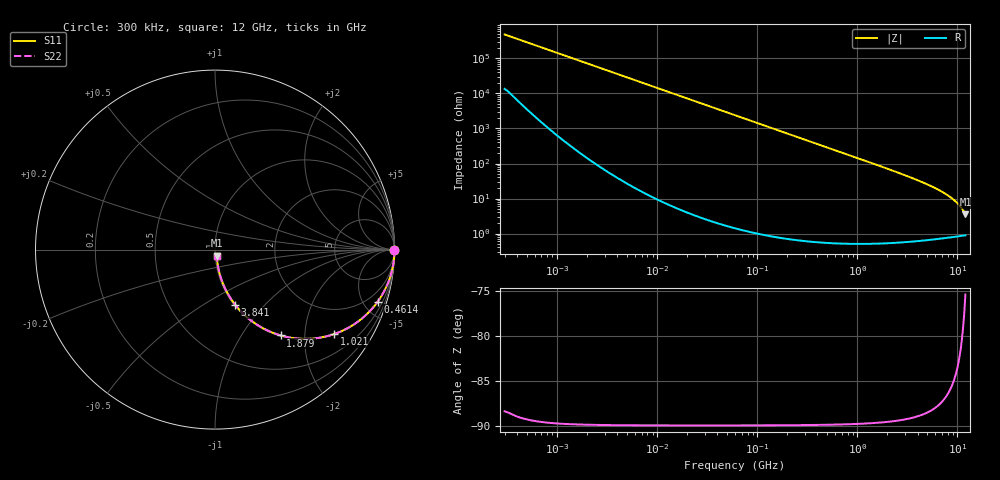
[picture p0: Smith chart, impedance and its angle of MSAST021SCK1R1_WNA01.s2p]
! MSAST021SCK1R1_WNA01  S-PARAMETER MODEL  ( General Type )
! Model Generated by TAIYO YUDEN Corporation (http://www.ty-top.com)
! Version 2.0
! TAIYO YUDEN Control No. 181101
! Copyright(c) 2015 TAIYO YUDEN CO.,LTD. All Rights Reserved.
! Product Description (link to TY-COMPAS)
! https://ds.yuden.co.jp/TYCOMPAS/or/detail?pn=MSAST021SCK1R1BWNA01&u=M
! Products Name : Multilayer Ceramic Capacitors
! Characteristics :
!  Capacitance : 1.1 pF , Rated Voltage : 25V , TCC : CK / C0K
!  Case Size : 0.25 x 0.125 / 0.0098 x 0.0049 [mm/inch] , Thickness : 0.125 / 0.0049 [mm/inch]
!  (Conditions: Temperature = 25 degC , DC Bias Current/Voltage = 0A / 0V)
! External Node Assignments :
!  1  o---| |---o  2
! GND o---------o GND
! Frequency Range : 0.3MHz  -  12000MHz  [ 401 STEP ]
# MHz S RI R 50
! Freq[MHz].  S11 Real  S11 Imag  S21 Real  S21 Imag  S12 Real  S12 Imag  S22 Real  S22 Imag
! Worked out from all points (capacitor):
!   401 points, 300 kHz to 12 GHz, reference 50 ohm
!   read as one part in series: C = 1.1 pF near 316.3 kHz
!   lowest |Z| = 3.54 ohm at 12 GHz (marker M1)
!   S11 on the Smith chart (normalised r, x): 300 kHz: open; 461.4 MHz: 1.01, -6.27; 1.021 GHz: 1.01, -2.82; 1.879 GHz: 1.01, -1.51; 3.841 GHz: 1.01, -0.70; 12 GHz: 1.02, -0.07
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0.3  1 -0.000207  5.83e-06 0.000207  5.83e-06 0.000207  1 -0.000207
1.769972  1 -0.00122  4.23e-06 0.00122  4.23e-06 0.00122  1 -0.00122
10.44266  0.9999 -0.00722  5.67e-05 0.00722  5.67e-05 0.00722  0.9999 -0.00722
60  0.9983 -0.0414  0.00174 0.0414  0.00174 0.0414  0.9983 -0.0414
159.8975  0.9878 -0.1092  0.0122 0.1092  0.0122 0.1092  0.9878 -0.1092
237.9135  0.9735 -0.1601  0.0265 0.1601  0.0265 0.1601  0.9735 -0.1601
353.9943  0.9432 -0.2308  0.0568 0.2308  0.0568 0.2308  0.9432 -0.2308
461.3684  0.9071 -0.2894  0.0929 0.2894  0.0929 0.2894  0.9071 -0.2894
686.4755  0.8149 -0.3871  0.1851 0.3871  0.1851 0.3871  0.8149 -0.3871
1021.415  0.6645 -0.4704  0.3355 0.4704  0.3355 0.4704  0.6645 -0.4704
1403.667  0.5102 -0.4974  0.4898 0.4974  0.4898 0.4974  0.5102 -0.4974
1878.541  0.365 -0.478  0.635 0.478  0.635 0.478  0.365 -0.478
2088.533  0.3161 -0.4611  0.6839 0.4611  0.6839 0.4611  0.3161 -0.4611
2870.14  0.1923 -0.3883  0.8077 0.3883  0.8077 0.3883  0.1923 -0.3883
3841.137  0.1128 -0.3078  0.8872 0.3078  0.8872 0.3078  0.1128 -0.3078
5715.274  0.0489 -0.2003  0.9511 0.2003  0.9511 0.2003  0.0489 -0.2003
7854.144  0.0232 -0.1239  0.9768 0.1239  0.9768 0.1239  0.0232 -0.1239
8732.115  0.018 -0.1003  0.982 0.1003  0.982 0.1003  0.018 -0.1003
9708.23  0.0142 -0.0775  0.9858 0.0775  0.9858 0.0775  0.0142 -0.0775
10511.28  0.0121 -0.0608  0.9879 0.0608  0.9879 0.0608  0.0121 -0.0608
11380.75  0.0106 -0.0444  0.9894 0.0444  0.9894 0.0444  0.0106 -0.0444
12000  0.00998 -0.0337  0.99 0.0337  0.99 0.0337  0.00998 -0.0337
